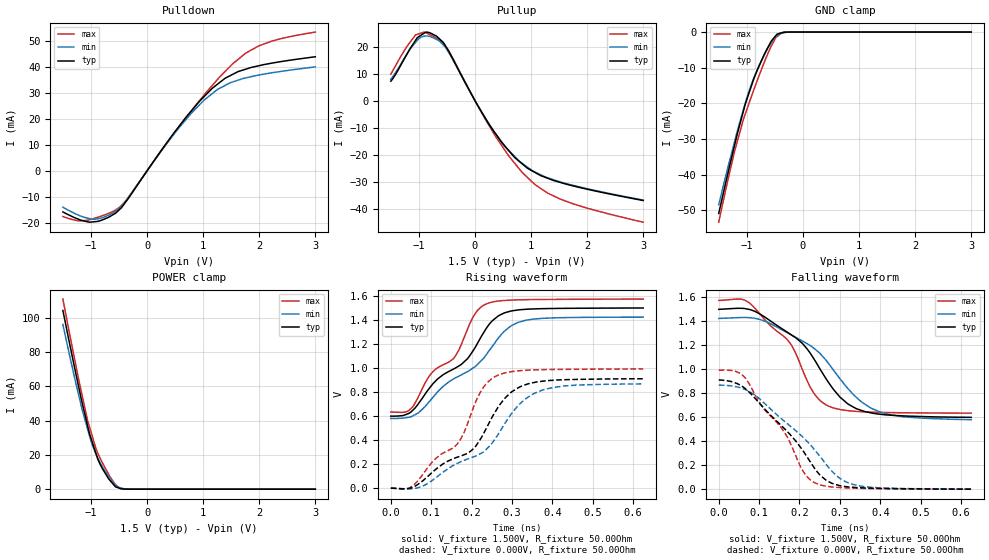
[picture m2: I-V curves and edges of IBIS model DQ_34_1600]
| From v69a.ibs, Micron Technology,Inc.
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| MODEL DQ_34_1600 (34 Ohm Data I/O with no ODT, 1600Mbps)
[Model]   DQ_34_1600
Model_type   I/O
Vinl = 600.000mV
Vinh = 900.000mV
Vmeas = 750.000mV
Vref = 750.000mV
Cref = 0.0pF
Rref = 25.000Ohm
|   typ   min   max
C_comp   1.24pF   1.09pF   1.39pF
[Model Spec]
| Input threshold voltage corners
Vinl   0.6000V   0.5625V   0.6375V
Vinh   0.9000V   0.8625V   0.9375V
| Measurement voltage corners
Vmeas   0.7500V   0.7125V   0.7875V
| Timing spec test load voltage corners
Vref   0.7500V   0.7125V   0.7875V
[Receiver Thresholds]
Vth   =  0.750V
Vth_min  =  0.735V
Vth_max  =  0.765V
Vinh_ac  =  0.150V
Vinh_dc  =  0.100V
Vinl_ac  = -0.150V
Vinl_dc  = -0.100V
Tslew_ac =  5.000ns |Not specified, so set to high value
Threshold_sensitivity = 0.50
Reference_supply Pullup_ref
[Voltage Range]   1.5000V   1.4250V   1.5750V
[Pullup Reference]   1.5000V   1.4250V   1.5750V
| Junction Temperature (Ambient temp is 35C typ, 95C min, 0C max)
[Temperature Range]   50.0   110.0   0.0
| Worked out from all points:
|   slope of the pulldown table from 0 to 0.225 V, typ, clamps not added: 31.9 ohm
|   slope of the pullup table from 0 to 0.225 V, typ, clamps not added: 28.4 ohm
|   GND clamp passes 1 mA (typ) near -0.48 V on its own axis
|   POWER clamp passes 1 mA (typ) near -0.53 V on its own axis
|   falling waveform, V_fixture 1.500V, R_fixture 50.00Ohm: 20-80 % time 132ps typ, 150ps min, 110ps max; typ from 1.5 V to 0.599 V
|   rising waveform, V_fixture 1.500V, R_fixture 50.00Ohm: 20-80 % time 150ps typ, 165ps min, 121ps max; typ from 0.599 V to 1.5 V
|   rising waveform, V_fixture 0.000V, R_fixture 50.00Ohm: 20-80 % time 156ps typ, 170ps min, 123ps max; typ from 0 V to 0.911 V
|   falling waveform, V_fixture 0.000V, R_fixture 50.00Ohm: 20-80 % time 138ps typ, 154ps min, 112ps max; typ from 0.911 V to 0 V
[Pulldown]
|   Voltage   I(typ)   I(min)   I(max)
-1.5V     -15.86mA   -14.03mA   -17.64mA
-1.22V    -18.7mA    -17.12mA   -19.3mA
-965mV    -19.7mA    -18.66mA   -18.5mA
-565mV    -16.41mA   -15.64mA   -15.16mA
-375mV    -11.88mA   -11.57mA   -11.45mA
340mV     10.5mA     10.24mA    10.27mA
795mV     23.28mA    22.39mA    23.33mA
1.025V    28.85mA    27.46mA    29.51mA
1.395V    35.82mA    33.03mA    38.47mA
1.755V    39.25mA    35.89mA    45.39mA
1.99V     40.6mA     37mA       48.26mA
3V        44.07mA    40.17mA    53.61mA
[GND Clamp]
|   Voltage   I(typ)   I(min)   I(max)
-1.5V     -50.86mA   -48.39mA   -53.31mA
-1.335V   -39.51mA   -37.89mA   -41.36mA
-1.22V    -31.91mA   -30.85mA   -33.59mA
-1.06V    -22.14mA   -21.75mA   -24.46mA
-1.03V    -20.37mA   -20.11mA   -23.1mA
-875mV    -13.13mA   -12.88mA   -16.2mA
-765mV    -8.986mA   -8.82mA    -11.56mA
-635mV    -4.662mA   -4.732mA   -6.435mA
-565mV    -2.562mA   -2.983mA   -3.942mA
-485mV    -1.053mA   -1.384mA   -1.64mA
-380mV    -208.9uA   -292.7uA   -211uA
3V        0A         0A         0A
[Pullup]
|   Voltage   I(typ)   I(min)   I(max)
-1.5V     7.178mA    7.94mA     9.786mA
-1.06V    22.29mA    21.51mA    24.28mA
-965mV    24.15mA    23.45mA    24.95mA
-800mV    25.06mA    23.7mA     24.38mA
-630mV    22.8mA     22.01mA    22.38mA
-485mV    18.85mA    18.42mA    19.1mA
245mV     -8.61mA    -8.358mA   -8.964mA
565mV     -17.63mA   -17.57mA   -19.3mA
935mV     -25mA      -24.59mA   -28.39mA
1.3V      -28.74mA   -28.56mA   -34.25mA
1.525V    -30.28mA   -30.1mA    -36.46mA
3V        -36.95mA   -36.79mA   -44.97mA
[POWER Clamp]
|   Voltage   I(typ)   I(min)   I(max)
-1.5V     104.2mA    96.04mA    110.8mA
-1.22V    59.88mA    55.04mA    64.17mA
-1.155V   50.11mA    46.13mA    54.38mA
-1.06V    36.99mA    35.03mA    40.06mA
-1.025V   32.28mA    30.95mA    36.2mA
-905mV    20.23mA    20.1mA     23.06mA
-800mV    12.24mA    13.34mA    15.7mA
-635mV    4.119mA    4.874mA    6.02mA
-565mV    1.438mA    2.643mA    2.719mA
-490mV    520.5uA    937.2uA    712uA
-285mV    1.423uA    9.711uA    221nA
3V        0A         0A         0A
[Ramp]
R_load = 50.00Ohm
|   typ   min   max
dV/dt_r   546.393mV/156.397ps 520.588mV/170.034ps 595.210mV/122.997ps
dV/dt_f   540.353mV/132.270ps 506.534mV/149.759ps 564.059mV/110.162ps
[Falling Waveform]
V_fixture = 1.500V
V_fixture_min = 1.425V
V_fixture_max = 1.575V
R_fixture = 50.00Ohm
|   Time   V(typ)   V(min)   V(max)
0s        1.5V       1.424V     1.574V
55ps      1.508V     1.432V     1.586V
80ps      1.495V     1.429V     1.542V
170ps     1.309V     1.304V     1.247V
205ps     1.223V     1.24V      1.016V
235ps     1.091V     1.177V     803.7mV
270ps     899.5mV    1.057V     695.9mV
320ps     710.4mV    839.2mV    654.8mV
400ps     624.9mV    643.4mV    640.4mV
625ps     599.3mV    579.8mV    634mV
[Rising Waveform]
V_fixture = 1.500V
V_fixture_min = 1.425V
V_fixture_max = 1.575V
R_fixture = 50.00Ohm
|   Time   V(typ)   V(min)   V(max)
0s        599.3mV    579.8mV    634mV
55ps      650.3mV    602.5mV    679.2mV
100ps     851.2mV    739mV      953.1mV
155ps     990.8mV    908.5mV    1.077V
190ps     1.078V     969.7mV    1.324V
215ps     1.208V     1.031V     1.481V
235ps     1.322V     1.105V     1.531V
280ps     1.457V     1.303V     1.562V
330ps     1.488V     1.394V     1.569V
625ps     1.5V       1.424V     1.574V
[Rising Waveform]
V_fixture = 0.000V
V_fixture_min = 0.000V
V_fixture_max = 0.000V
R_fixture = 50.00Ohm
|   Time   V(typ)   V(min)   V(max)
0s        -4.765uV   270.2uV    159.9uV
55ps      8.779mV    -3.827mV   19.75mV
110ps     152.5mV    82.57mV    242.2mV
165ps     257.8mV    206.4mV    369.3mV
205ps     328.7mV    260.5mV    676.1mV
225ps     424.7mV    292.7mV    818.2mV
265ps     671mV      443.1mV    939.8mV
315ps     833.9mV    687.1mV    976.2mV
375ps     889.9mV    815.6mV    986.2mV
625ps     910.7mV    867.9mV    992.2mV
[Falling Waveform]
V_fixture = 0.000V
V_fixture_min = 0.000V
V_fixture_max = 0.000V
R_fixture = 50.00Ohm
|   Time   V(typ)   V(min)   V(max)
0s        910.7mV    867.9mV    992.2mV
40ps      887.4mV    856.4mV    984.3mV
65ps      840.6mV    832.4mV    930.6mV
110ps     682.4mV    726.7mV    678.7mV
165ps     497.1mV    559.9mV    461.8mV
215ps     288.1mV    411.7mV    117.8mV
240ps     161.5mV    318mV      49.88mV
295ps     33.6mV     103.4mV    14.44mV
335ps     14.87mV    37.3mV     8.162mV
625ps     -4.765uV   270.2uV    159.9uV
